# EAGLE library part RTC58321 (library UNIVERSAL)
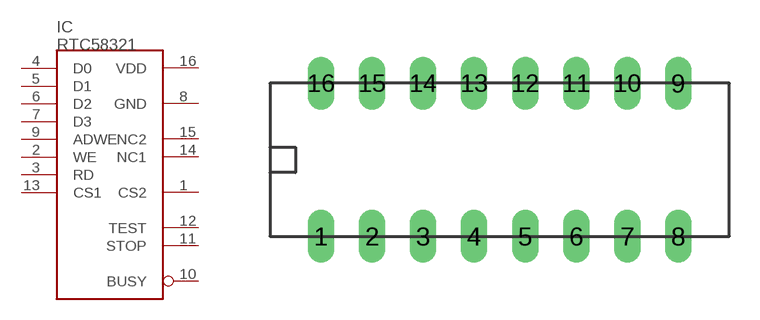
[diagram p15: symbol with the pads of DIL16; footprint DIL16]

Designator prefix IC

## RTC58321  [DIL16]
1  CS2  in
2  WE  in
3  RD  in
4  D0  in
5  D1  in
6  D2  in
7  D3  in
8  GND  pwr
9  ADWE  in
10  BUSY  out
11  STOP  in
12  TEST  in
13  CS1  in
14  NC1  nc
15  NC2  nc
16  VDD  sup

## Footprint DIL16 (pad centres in mm)
drill 0.813 pad 1.27 long: 1 0,1.27; 2 2.54,1.27; 3 5.08,1.27; 4 7.62,1.27; 5 10.16,1.27; 6 12.7,1.27; 7 15.24,1.27; 8 17.78,1.27; 9 17.78,8.89; 10 15.24,8.89; 11 12.7,8.89; 12 10.16,8.89; 13 7.62,8.89; 14 5.08,8.89; 15 2.54,8.89; 16 0,8.89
